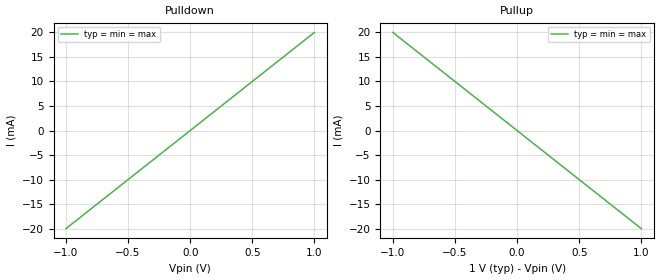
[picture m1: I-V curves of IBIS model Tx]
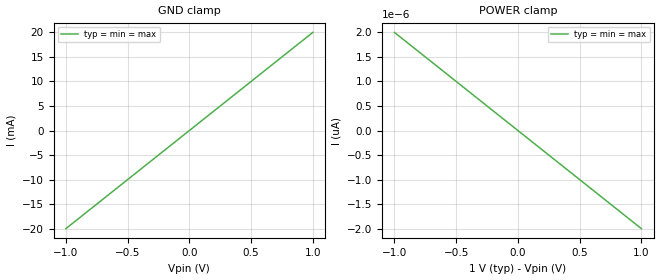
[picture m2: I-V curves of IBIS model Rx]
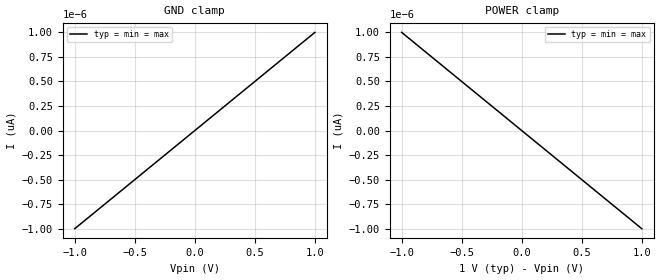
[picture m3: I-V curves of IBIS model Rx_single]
[IBIS Ver]   5.0
[File Name]  ibis.ibs
[File Rev]   1.0
[Notes]   Default IBIS file for Topology Explorer
[Disclaimer] Template model only
|   COMPONENT: Default
[Component] Default
[Manufacturer] Cadence Design Systems, Inc.
[Package]
| variable typ   min max
R_pkg   0.1m  NA  NA
L_pkg   0.1nH NA  NA
C_pkg   1.0pF NA  NA
[Pin] signal_name model_name R_pin L_pin C_pin
1   TX_P   Tx
2   TX_N   Tx
3   RX_P   Rx
4   RX_N   Rx
5   TX   Tx
6   RX   Rx_single
7   POWER   POWER
8   GND   GND
[Pin Mapping]   pulldown_ref   pullup_ref  gnd_clamp_ref   power_clamp_ref
1   gndbus   pwrbus
2   gndbus   pwrbus
3   gndbus   pwrbus
4   gndbus   pwrbus
5   gndbus   pwrbus
6   gndbus   pwrbus
7   NC   pwrbus
8   gndbus   NC
[Diff Pin] inv_pin vdiff  tdelay_typ tdelay_min tdelay_max
1   2   25mV   NA   NA   NA
3   4   25mV   NA   NA   NA
| Models and submodels in the file (3): Tx (Output), Rx (Input), Rx_single (Input)
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[Model] Tx
Model_type Output
Vmeas = 500.000mV
Vref = 500.000mV
Cref = 0.0pF
Rref = 50.000Ohm
| variable typ min max
C_comp   0.1pF 0.1pF   0.1pF
[Voltage Range] 1.0 1.0 1.0
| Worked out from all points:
|   slope of the pulldown table from 0 to 0.15 V, typ, clamps not added: 50 ohm
|   slope of the pullup table from 0 to 0.15 V, typ, clamps not added: 50 ohm
[Pullup]
-1V       20mA       20mA       20mA
0V        0A         0A         0A
1V        -20mA      -20mA      -20mA
[Pulldown]
-1V       -20mA      -20mA      -20mA
0V        0A         0A         0A
1V        20mA       20mA       20mA
[Ramp]
 dV/dt_r  0.32/25ps NA NA
 dV/dt_f  0.32/25ps NA NA
R_load = 50
[Model] Rx
Model_type Input
Vinl=-0.2V
Vinh=0.2V
| variable typ min max
C_comp   0.1pF 0.1pF 0.1pF
[Voltage Range] 1.0 1.0 1.0
[POWER_clamp]
|voltage I(typ)
-1V       2pA        2pA        2pA
0V        0A         0A         0A
1V        -2pA       -2pA       -2pA
[GND_clamp]
|voltage I(typ)
-1V       -20mA      -20mA      -20mA
0V        0A         0A         0A
1V        20mA       20mA       20mA
[Model] Rx_single
Model_type Input
Vinl=0.4V
Vinh=0.6V
| variable typ min max
C_comp   0.1pF 0.1pF 0.1pF
[Voltage Range] 1.0 1.0 1.0
[POWER_clamp]
|voltage I(typ)
-1V       1pA        1pA        1pA
0V        0A         0A         0A
1V        -1pA       -1pA       -1pA
[GND_clamp]
|voltage I(typ)
-1V       -1pA       -1pA       -1pA
0V        0A         0A         0A
1V        1pA        1pA        1pA
